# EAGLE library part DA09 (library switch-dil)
DIL/CODE SWITCH
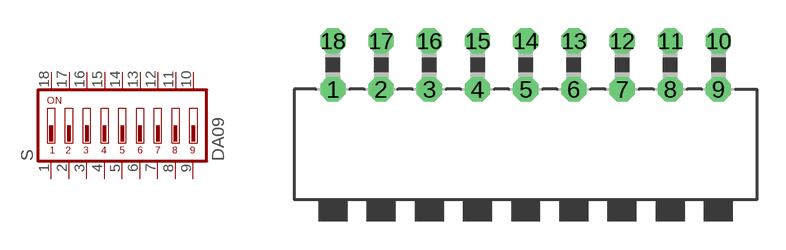
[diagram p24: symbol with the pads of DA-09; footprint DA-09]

Designator prefix S

## DA09 (MPN: MCDA09; OC_FARNELL: 1522003; OC_NEWARK: 74M2975)  [DA-09]
1  1  pas
2  2  pas
3  3  pas
4  4  pas
5  5  pas
6  6  pas
7  7  pas
8  8  pas
9  9  pas
10  10  pas
11  11  pas
12  12  pas
13  13  pas
14  14  pas
15  15  pas
16  16  pas
17  17  pas
18  18  pas

## Footprint DA-09 (pad centres in mm)
DIL/CODE SWITCH Mors
drill 0.813 octagon: 1 -10.16,-1.27; 2 -7.62,-1.27; 3 -5.08,-1.27; 4 -2.54,-1.27; 5 0,-1.27; 6 2.54,-1.27; 7 5.08,-1.27; 8 7.62,-1.27; 9 10.16,-1.27; 10 10.16,1.27; 11 7.62,1.27; 12 5.08,1.27; 13 2.54,1.27; 14 0,1.27; 15 -2.54,1.27; 16 -5.08,1.27; 17 -7.62,1.27; 18 -10.16,1.27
